FUNCTION_BLOCK motor
VAR_INPUT
	vrtiNaprej: BOOL;
	vrtiNazaj: BOOL;
END_VAR
VAR_OUTPUT
	smer: BOOL;
	premik: BOOL;
END_VAR

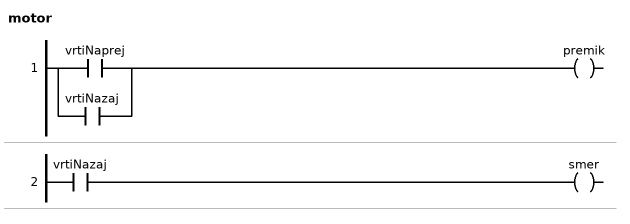
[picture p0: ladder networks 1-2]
// NETWORK 1
premik := vrtiNaprej OR vrtiNazaj;

// NETWORK 2
smer := vrtiNazaj;

END_FUNCTION_BLOCK
